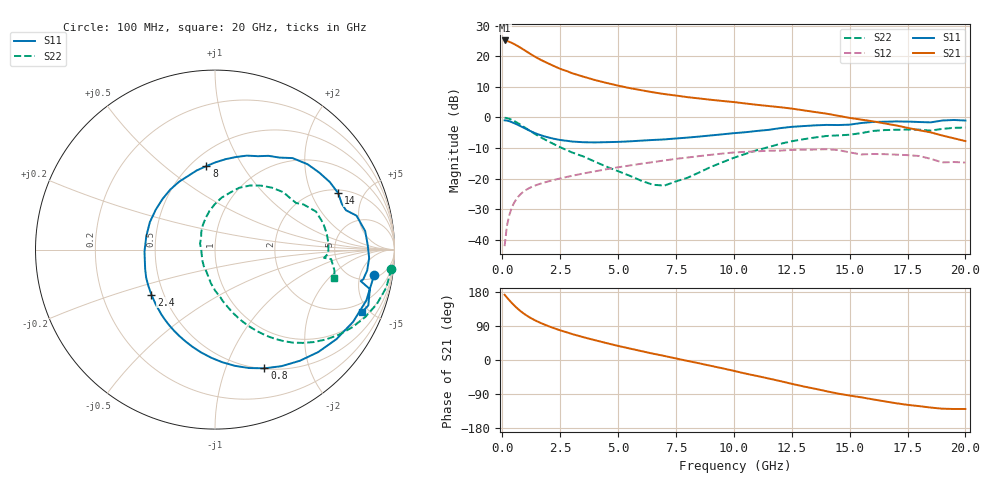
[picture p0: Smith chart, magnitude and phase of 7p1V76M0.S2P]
! Infineon Technologies  Discrete & RF Semiconductors
! bfp620
! VCE =  1.7 V,  IC =  6.0 mA
! Common Emitter S-Parameters:  Sep 2002
# GHz  S  MA  R  50
!  f  S11  S21  S12  S22
! GHz  MAG  ANG  MAG  ANG  MAG  ANG  MAG  ANG
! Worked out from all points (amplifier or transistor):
!   59 points, 100 MHz to 20 GHz, reference 50 ohm
!   highest |S21| = 25.2 dB at 100 MHz (marker M1)
!   |S21| within 3 dB of that: start of sweep to 919.9 MHz
!   unconditionally stable (mu >= 1): 4.649 GHz to 11.38 GHz; 14.89 GHz to 15.12 GHz; 17.12 GHz to end of sweep
!   at 1 GHz: K = 0.36, MSG = 22.8 dB, |S12| = -23.8 dB
!   at 5.5 GHz: K = 1.04, MAG = 11.4 dB, |S12| = -15.7 dB
!   at 20 GHz: K = 1.36, MAG = -0.1 dB, |S12| = -14.8 dB
!   S11 on the Smith chart (normalised r, x): 100 MHz: 6, -9; 800 MHz: 0.51, -1.37; 2.4 GHz: 0.43, -0.26; 8 GHz: 0.59, +0.71; 14 GHz: 2.18, +3.19; 20 GHz: 1.34, -4.49
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0.1  0.8974 -9.2  18.23 172.1  0.0078 81.5  0.989 -6.2
0.2  0.8896 -18.6  17.9 164.9  0.0168 80.2  0.977 -12.6
0.3  0.8684 -27.6  17.35 157.9  0.025 75.8  0.9514 -18.6
0.4  0.8407 -36.4  16.7 151.2  0.0326 71.4  0.9175 -24.2
0.5  0.8103 -44.8  15.99 144.9  0.0394 67.2  0.879 -29.5
0.6  0.779 -52.7  15.25 139.0  0.0455 63.5  0.8382 -34.4
0.8  0.7165 -67.4  13.78 128.4  0.0559 57.1  0.7551 -43.0
1.1  0.6285 -86.4  11.68 115.5  0.0676 49.8  0.6379 -53.1
1.3  0.5786 -97.6  10.48 108.4  0.0736 46.2  0.5702 -58.3
1.5  0.5381 -107.6  9.467 102.2  0.0788 43.4  0.5126 -62.6
1.9  0.4808 -125.2  7.941 91.6  0.0878 39.4  0.4234 -69.5
2.4  0.4342 -144.7  6.499 80.4  0.0982 35.7  0.3397 -76.4
3  0.4037 -164.6  5.327 68.8  0.1105 32.0  0.2681 -83.5
3.5  0.393 -178.4  4.656 60.2  0.121 29.0  0.2298 -89.6
5  0.398 146.0  3.321 37.2  0.1527 19.5  0.1318 -111.4
7  0.4369 110.0  2.416 10.7  0.1974 5.1  0.0766 -179.5
8  0.4677 95.9  2.149 -2.4  0.2205 -3.7  0.1029 138.8
10.5  0.5728 65.3  1.694 -35.8  0.2735 -29.2  0.253 90.3
13.5  0.7421 30.5  1.228 -75.8  0.2982 -61.0  0.4696 47.2
14  0.7549 24.6  1.154 -82.4  0.3017 -67.4  0.4973 40.0
17  0.86 -3.1  0.741 -114.0  0.2462 -91.7  0.629 8.1
20  0.8894 -23.2  0.41 -129.3  0.183 -105.0  0.6825 -13.4
